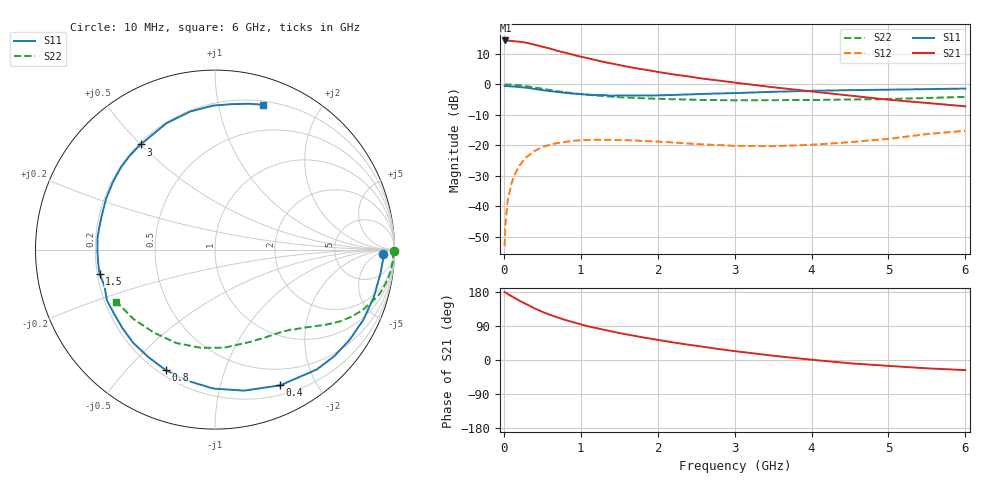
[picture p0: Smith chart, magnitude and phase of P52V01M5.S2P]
! SIEMENS Small Signal Semiconductors
! BFP183
! Si NPN RF Bipolar Junction Transistor in SOT143
! VCE = 2 V  IC = 1.5 mA
! Common Emitter S-Parameters:  March  1996
# GHz  S  MA  R  50
!  f  S11  S21  S12  S22
! GHz  MAG  ANG  MAG  ANG  MAG  ANG  MAG  ANG
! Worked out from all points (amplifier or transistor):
!   36 points, 10 MHz to 6 GHz, reference 50 ohm
!   highest |S21| = 14.4 dB at 20 MHz (marker M1)
!   |S21| within 3 dB of that: start of sweep to 645.6 MHz
!   unconditionally stable (mu >= 1): 2.245 GHz to end of sweep
!   at 250 MHz: K = 0.10, MSG = 19.5 dB, |S12| = -25.1 dB
!   at 1.4 GHz: K = 0.62, MSG = 12.5 dB, |S12| = -18.2 dB
!   at 6 GHz: K = 1.02, MAG = 3.1 dB, |S12| = -15.3 dB
!   S11 on the Smith chart (normalised r, x): 10 MHz: 27, -11; 400 MHz: 0.30, -1.55; 800 MHz: 0.23, -0.65; 1.5 GHz: 0.21, -0.10; 3 GHz: 0.21, +0.50; 6 GHz: 0.23, +1.36
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0.01  0.9382 -1.5  5.227 179.2  0.0022 84.7  0.9994 -0.6
0.02  0.938 -3.4  5.251 178.3  0.0049 89.0  0.9909 -1.2
0.05  0.9312 -8.4  5.219 174.2  0.0123 87.7  0.9945 -3.1
0.1  0.9235 -16.8  5.15 168.4  0.0237 80.1  0.9873 -6.3
0.15  0.9144 -25.4  5.077 162.6  0.0348 75.1  0.9779 -9.4
0.25  0.891 -41.9  4.909 151.4  0.0554 66.2  0.949 -15.2
0.3  0.8759 -49.7  4.798 146.6  0.0646 61.8  0.9271 -17.7
0.4  0.8391 -64.3  4.476 136.2  0.0806 53.7  0.8888 -22.3
0.5  0.8024 -78.3  4.151 127.1  0.093 46.3  0.8462 -26.3
0.6  0.7744 -90.7  3.873 119.3  0.1023 40.3  0.8063 -29.6
0.7  0.7464 -102.0  3.54 112.3  0.1088 35.1  0.7694 -32.3
0.8  0.7255 -112.2  3.299 105.6  0.1135 30.0  0.7391 -34.7
1  0.691 -131.4  2.839 94.1  0.1202 22.4  0.6899 -38.5
1.1  0.676 -139.9  2.669 88.7  0.1222 19.3  0.671 -40.1
1.5  0.6569 -168.2  2.077 71.2  0.1211 9.9  0.6147 -46.4
1.8  0.6578 174.1  1.766 59.9  0.1182 5.8  0.5904 -50.9
2.2  0.6694 155.1  1.458 46.4  0.1109 2.5  0.569 -57.6
3  0.7172 125.2  1.068 23.5  0.0976 4.7  0.5457 -73.6
3.5  0.7541 111.1  0.896 11.3  0.0964 10.3  0.5493 -84.9
4.5  0.8026 90.6  0.653 -8.7  0.1122 21.3  0.5635 -112.6
5.5  0.8334 77.1  0.494 -22.0  0.1525 23.8  0.5964 -139.4
6  0.8514 71.5  0.435 -26.7  0.1727 20.7  0.6215 -152.1
